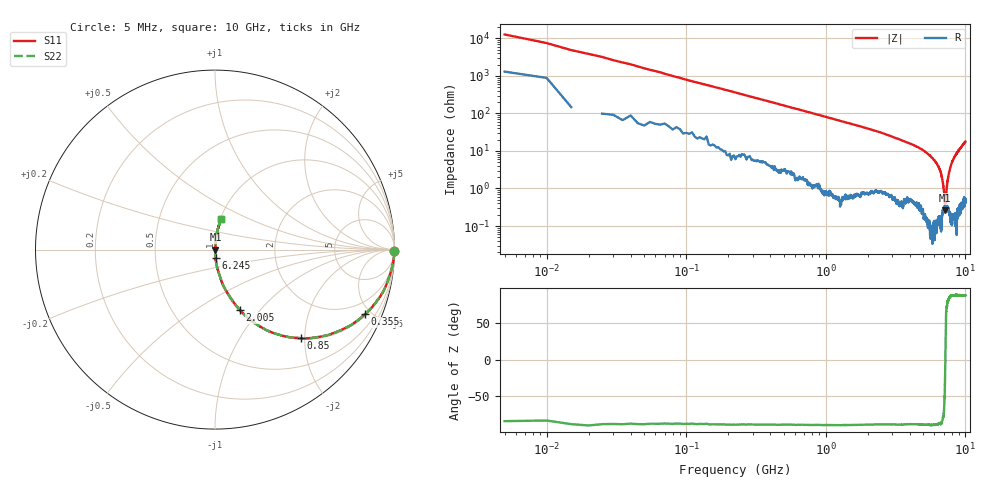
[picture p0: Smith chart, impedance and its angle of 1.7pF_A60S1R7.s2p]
! Amotech Co.,Ltd.
! http://www.amotech.co.kr/
! Part Number: A60S1R7
! These Parameters are Measured in Series Mode Connection
! Operation Temp=25[degC], DC Bias Voltage=0[V]
! Freq. Start=5[MHz] Stop=10[GHz], 2000[Steps]
! Date: Monday, July 13, 2020, 01:25:02
# GHZ S RI R 50.000000
!Freq.(Hz) S11(Real) S11(Imag) S21(Real) S21(Imag) S12(Real) S12(Imag) S22(Real) S22(Imag)
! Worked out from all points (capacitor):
!   2000 points, 5 MHz to 10 GHz, reference 50 ohm
!   read as one part in series: C = 2 pF near 55 MHz
!   lowest |Z| = 264 mohm at 7.17 GHz (marker M1)
!   series resonance near 7.183 GHz, so ESL is about 250 pH
!   S11 on the Smith chart (normalised r, x): 5 MHz: open; 355 MHz: 1.11, -4.58; 850 MHz: 1.02, -1.91; 2.005 GHz: 1.02, -0.79; 6.245 GHz: 1.00, -0.09; 10 GHz: 1.01, +0.36
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0.005  0.9991 -0.00783  0.000869 0.00783  0.000869 0.00783  0.9991 -0.00783
0.065  0.9905 -0.0791  0.00952 0.0791  0.00952 0.0791  0.9905 -0.0791
0.115  0.9747 -0.1406  0.0253 0.1406  0.0253 0.1406  0.9747 -0.1406
0.21  0.9344 -0.2401  0.0656 0.2401  0.0656 0.2401  0.9344 -0.2401
0.355  0.8344 -0.3604  0.1656 0.3604  0.1656 0.3604  0.8344 -0.3604
0.565  0.6724 -0.4595  0.3276 0.4595  0.3276 0.4595  0.6724 -0.4595
0.85  0.4779 -0.4934  0.5221 0.4934  0.5221 0.4934  0.4779 -0.4934
1.675  0.1887 -0.384  0.8113 0.384  0.8113 0.384  0.1887 -0.384
2.005  0.1391 -0.3366  0.8609 0.3366  0.8609 0.3366  0.1391 -0.3366
3.34  0.0433 -0.1944  0.9567 0.1944  0.9567 0.1944  0.0433 -0.1944
5.005  0.0125 -0.1013  0.9875 0.1013  0.9875 0.1013  0.0125 -0.1013
6.245  0.00297 -0.0456  0.997 0.0456  0.997 0.0456  0.00297 -0.0456
6.67  0.0019 -0.0266  0.9981 0.0266  0.9981 0.0266  0.0019 -0.0266
6.975  0.00251 -0.0104  0.9975 0.0104  0.9975 0.0104  0.00251 -0.0104
7.135  0.00261 -0.00178  0.9974 0.00178  0.9974 0.00178  0.00261 -0.00178
7.17  0.00263 -0.000162  0.9974 0.000162  0.9974 0.000162  0.00263 -0.000162
7.295  0.00308 0.00681  0.9969 -0.00681  0.9969 -0.00681  0.00308 0.00681
7.39  0.00329 0.0117  0.9967 -0.0117  0.9967 -0.0117  0.00329 0.0117
7.61  0.00314 0.0248  0.9969 -0.0248  0.9969 -0.0248  0.00314 0.0248
7.925  0.0039 0.045  0.9961 -0.045  0.9961 -0.045  0.0039 0.045
8.335  0.00614 0.0671  0.9939 -0.0671  0.9939 -0.0671  0.00614 0.0671
10  0.035 0.1715  0.965 -0.1715  0.965 -0.1715  0.035 0.1715
